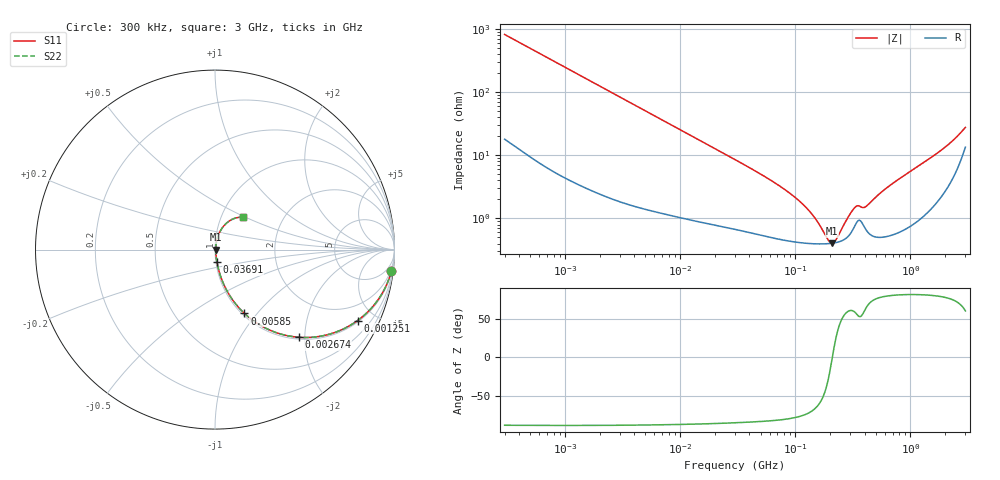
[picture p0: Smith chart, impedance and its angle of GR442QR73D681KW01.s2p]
!Murata Part Number: GR442QR73D681KW01
!These Parameters are Measured in Series Mode Connection
!Data Generated on Mar 13, 2026
!  o--ll--o
!Port1  Port2
!  o------o
!Operation Temp=25[degC], DC Bias Voltage=0[V]
!Freq. Start=300[kHz] Stop=3[GHz] 401[Steps]
# Hz S RI R 50
!Freq.(Hz) S11(Real) S11(Imag) S21(Real) S21(Imag) S12(Real) S12(Imag) S22(Real) S22(Imag)
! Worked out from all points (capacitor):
!   401 points, 300 kHz to 3 GHz, reference 50 ohm
!   read as one part in series: C = 646 pF near 314.1 kHz
!   lowest |Z| = 404 mohm at 207.5 MHz (marker M1)
!   series resonance near 209.9 MHz, so ESL is about 890 pH
!   S11 on the Smith chart (normalised r, x): 300 kHz: 1, -16; 1.251 MHz: 1.07, -3.98; 2.674 MHz: 1.04, -1.87; 5.85 MHz: 1.03, -0.86; 36.91 MHz: 1.01, -0.14; 3 GHz: 1.27, +0.48
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300000  0.9827 -0.1198  0.0173 0.1198  0.0173 0.1198  0.9827 -0.1198
687260  0.9246 -0.2552  0.0754 0.2552  0.0754 0.2552  0.9246 -0.2552
1250608  0.7942 -0.3955  0.2058 0.3955  0.2058 0.3955  0.7942 -0.3955
1403205  0.7551 -0.421  0.2449 0.421  0.2449 0.421  0.7551 -0.421
2673753  0.4679 -0.4885  0.5321 0.4885  0.5321 0.4885  0.4679 -0.4885
4046889  0.2831 -0.4382  0.7169 0.4382  0.7169 0.4382  0.2831 -0.4382
5849534  0.1641 -0.3556  0.8359 0.3556  0.8359 0.3556  0.1641 -0.3556
6563285  0.1367 -0.3279  0.8633 0.3279  0.8633 0.3279  0.1367 -0.3279
1.222141e7  0.0497 -0.1958  0.9503 0.1958  0.9503 0.1958  0.0497 -0.1958
3e7  0.0137 -0.0834  0.9863 0.0834  0.9863 0.0834  0.0137 -0.0834
3.690806e7  0.0108 -0.0677  0.9892 0.0677  0.9892 0.0677  0.0108 -0.0677
8.652094e7  0.00504 -0.0257  0.995 0.0257  0.995 0.0257  0.00504 -0.0257
1.403205e8  0.00407 -0.0108  0.9959 0.0108  0.9959 0.0108  0.00407 -0.0108
1.936963e8  0.00397 -0.00214  0.996 0.00214  0.996 0.00214  0.00397 -0.00214
2.075493e8  0.00401 -0.000303  0.996 0.000303  0.996 0.000303  0.00401 -0.000303
2.275733e8  0.00413 0.00218  0.9959 -0.00218  0.9959 -0.00218  0.00413 0.00218
2.864978e8  0.00519 0.00885  0.9948 -0.00885  0.9948 -0.00885  0.00519 0.00885
3.289435e8  0.0077 0.0126  0.9923 -0.0126  0.9923 -0.0126  0.0077 0.0126
4.141153e8  0.00665 0.014  0.9934 -0.014  0.9934 -0.014  0.00665 0.014
6.563285e8  0.00628 0.0319  0.9937 -0.0319  0.9937 -0.0319  0.00628 0.0319
1.892872e9  0.0363 0.1148  0.9637 -0.1148  0.9637 -0.1148  0.0363 0.1148
3e9  0.1563 0.1791  0.8437 -0.1791  0.8437 -0.1791  0.1563 0.1791
